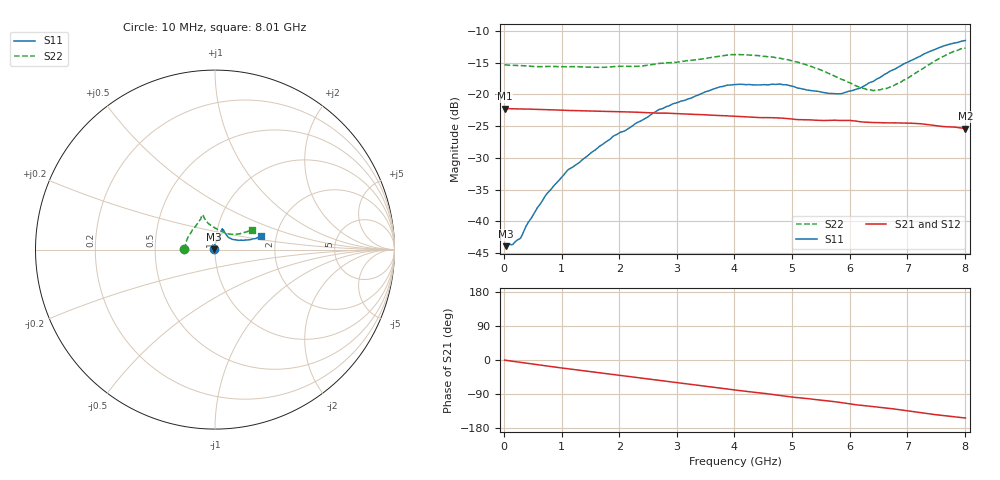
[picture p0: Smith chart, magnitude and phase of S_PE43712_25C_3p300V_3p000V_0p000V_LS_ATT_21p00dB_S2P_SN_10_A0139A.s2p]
! DEVICE ID: PE43712
! File Path: z:\PE43713\PE43713_CHAR_NOM_04292014\AMB\3p300\LS_ATT_21p00dB\PE43713_AMB_3p300V_3p000V_0p000V_LS_ATT_21p00dB_S2P_SN_10_A0139A.s2p
! Serial: 10
! Lot: A0139A
! Temp: 25C
! VDD: 3.300
! VSS: 0.000
! Control_Hi: 3.000
! Control_Lo: 0.000
! Attenuation Step: 21.00dB
! Port 1: RF1
! Port 2: RF2
! ThroughPath:1-2
! IDD: 0.0001470956
! ISS: -1.694e-007
#  Hz  S  RI  R  50
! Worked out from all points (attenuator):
!   801 points, 10 MHz to 8.01 GHz, reference 50 ohm
!   highest |S21| = -22.23 dB at 10 MHz (marker M1); lowest = -25.4 dB at 8.01 GHz (marker M2)
!   lowest |S11| = -43.9 dB at 30 MHz (marker M3), VSWR 1.01, Z = 49.4 + j0.135 ohm
!   |S11| at or under -10 dB: start of sweep to end of sweep
!   |S22| runs from -19.4 to -12.7 dB; largest |S21 - S12| = 0.00029
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1e7  -0.0066 0.000574  0.0773 -0.000395  0.0773 -0.000366  -0.1715 0.00121
3e7  -0.00621 0.00137  0.0773 -0.000958  0.0773 -0.000976  -0.1709 0.00283
1.5e8  -0.0054 0.00376  0.077 -0.00453  0.077 -0.00453  -0.1694 0.0105
2.8e8  -0.00458 0.00572  0.0764 -0.00825  0.0764 -0.0083  -0.1676 0.0172
4.2e8  -0.00435 0.00877  0.0757 -0.0122  0.0756 -0.0122  -0.1657 0.0245
7.4e8  -0.004 0.0159  0.073 -0.0206  0.073 -0.0206  -0.1607 0.0429
1.1e9  -0.00254 0.0251  0.0689 -0.0292  0.069 -0.0292  -0.1534 0.062
1.35e9  -6.27e-05 0.0303  0.0658 -0.0347  0.0658 -0.0347  -0.1475 0.0734
1.91e9  0.00872 0.0464  0.0572 -0.0458  0.0572 -0.0458  -0.1294 0.1037
2.68e9  0.0269 0.0706  0.0424 -0.0573  0.0423 -0.0573  -0.0989 0.1449
3.72e9  0.0389 0.1069  0.0192 -0.0655  0.0191 -0.0655  -0.0755 0.1846
4.01e9  0.0403 0.1128  0.0127 -0.0661  0.0127 -0.0661  -0.0751 0.1923
4.79e9  0.044 0.1124  -0.00398 -0.065  -0.00399 -0.0651  -0.0636 0.1824
5.35e9  0.0565 0.0908  -0.0146 -0.0612  -0.0146 -0.0612  -0.0496 0.1577
5.87e9  0.0771 0.0664  -0.0241 -0.0576  -0.024 -0.0575  -0.0149 0.1303
6.17e9  0.0954 0.0577  -0.0298 -0.0533  -0.0296 -0.0533  0.0128 0.1129
6.38e9  0.1125 0.0553  -0.0321 -0.0507  -0.032 -0.0507  0.0357 0.1018
6.68e9  0.1414 0.0518  -0.0363 -0.0473  -0.0362 -0.0473  0.0707 0.0888
7e9  0.1706 0.0533  -0.0412 -0.0428  -0.0411 -0.0428  0.1033 0.0846
7.55e9  0.2252 0.0623  -0.0463 -0.032  -0.0463 -0.032  0.1657 0.0961
7.81e9  0.2442 0.0698  -0.0477 -0.028  -0.0477 -0.028  0.1914 0.1057
8.01e9  0.2554 0.076  -0.048 -0.0245  -0.0478 -0.0246  0.2038 0.1099
